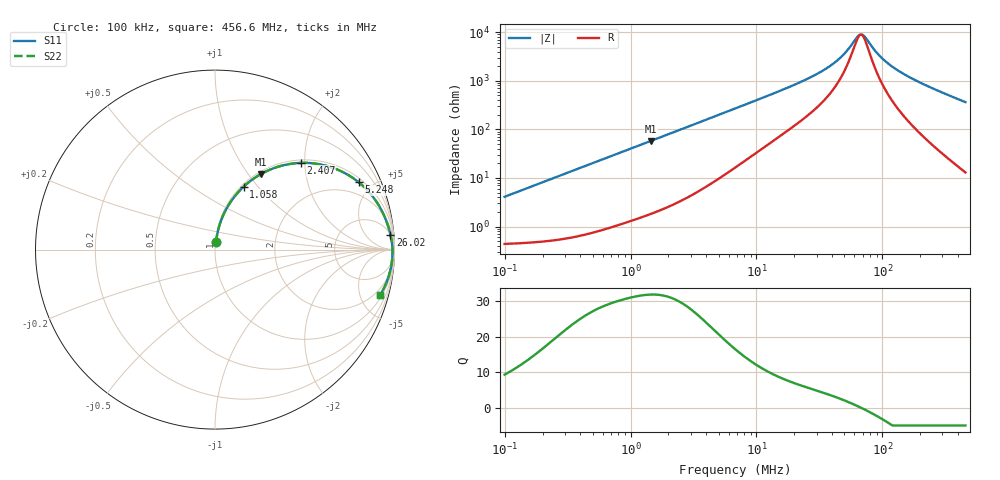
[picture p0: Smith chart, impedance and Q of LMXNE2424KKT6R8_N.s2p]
! LMXNE2424KKT6R8_N  S-PARAMETER MODEL  ( General Type )
! Model Generated by TAIYO YUDEN Corporation (https://www.yuden.co.jp/en/)
! Version 1.0
! TAIYO YUDEN Control No. 191023NI43SB-FBB
! Copyright(c) 2019 TAIYO YUDEN CO.,LTD. All Rights Reserved.
! Product Description (link to TY-COMPAS)
! https://ds.yuden.co.jp/TYCOMPAS/or/detail?pn=LMXNE2424KKT6R8MN&u=M
! Products Name : Inductors
! Characteristics :
!  Inductance : 6.8 uH , SRF(min) : 43 MHz , DC Resistance(max) : 0.492 Ohm
!  Rated Current : Saturation :750 mA , Temp Rise : 570 mA (40 degC)
!  Case Size : 2.4 x 2.4 / 0.095 x 0.095 [mm/inch] , Thickness : 1 / 0.039 [mm/inch]
!  (Conditions: Temperature = 25 degC , DC Bias Current/Voltage = 0A / 0V)
! External Node Assignments :
!  1  o---GGG---o  2
! GND o---------o GND
! Frequency Range : 0.1MHz  -  456.598367MHz  [ 402 STEP ]
# MHz S RI R 50
! Freq[MHz].  S11 Real  S11 Imag  S21 Real  S21 Imag  S12 Real  S12 Imag  S22 Real  S22 Imag
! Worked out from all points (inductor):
!   401 points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, 100 kHz to 456.6 MHz, reference 50 ohm
!   read as one part in series: L = 6.47 uH near 104.3 kHz
!   highest Q = 31.8 at 1.452 MHz (marker M1), where L = 6.34 uH
!   self-resonance near 67.14 MHz
!   S11 on the Smith chart (normalised r, x): 100 kHz: 1.01, +0.08; 1.058 MHz: 1.03, +0.85; 2.407 MHz: 1.06, +1.91; 5.248 MHz: 1.21, +4.15; 26.02 MHz: 5, +22; 456.6 MHz: 1.26, -7.27
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0.1  0.006 0.0403  0.994 -0.0403  0.994 -0.0403  0.006 0.0403
0.410178  0.0327 0.1593  0.9673 -0.1593  0.9673 -0.1593  0.0327 0.1593
0.694533  0.0797 0.2544  0.9203 -0.2544  0.9203 -0.2544  0.0797 0.2544
1.058448  0.1597 0.3506  0.8403 -0.3506  0.8403 -0.3506  0.1597 0.3506
1.451785  0.2572 0.4216  0.7428 -0.4216  0.7428 -0.4216  0.2572 0.4216
1.682457  0.3147 0.4489  0.6853 -0.4489  0.6853 -0.4489  0.3147 0.4489
2.40699  0.4777 0.4831  0.5223 -0.4831  0.5223 -0.4831  0.4777 0.4831
3.443534  0.6452 0.4596  0.3548 -0.4596  0.3548 -0.4596  0.6452 0.4596
5.247847  0.8003 0.3755  0.1997 -0.3755  0.1997 -0.3755  0.8003 0.3755
6.901063  0.8675 0.3096  0.1325 -0.3096  0.1325 -0.3096  0.8675 0.3096
11.93399  0.9408 0.1927  0.0592 -0.1927  0.0592 -0.1927  0.9408 0.1927
26.01912  0.9773 0.0839  0.0227 -0.0839  0.0227 -0.0839  0.9773 0.0839
27.71655  0.9788 0.0773  0.0212 -0.0773  0.0212 -0.0773  0.9788 0.0773
44.05686  0.9862 0.0347  0.0138 -0.0347  0.0138 -0.0347  0.9862 0.0347
52.14399  0.9877 0.0208  0.0123 -0.0208  0.0123 -0.0208  0.9877 0.0208
63.02949  0.9888 0.0055  0.0112 -0.0055  0.0112 -0.0055  0.9888 0.0055
67.14138  0.989 0.000441  0.011 -0.000441  0.011 -0.000441  0.989 0.000441
73.04418  0.9892 -0.00634  0.0108 0.00634  0.0108 0.00634  0.9892 -0.00634
92.0922  0.989 -0.0255  0.011 0.0255  0.011 0.0255  0.989 -0.0255
113.6871  0.988 -0.0441  0.012 0.0441  0.012 0.0441  0.988 -0.0441
196.5988  0.9794 -0.1034  0.0206 0.1034  0.0206 0.1034  0.9794 -0.1034
456.5984  0.922 -0.251  0.078 0.251  0.078 0.251  0.922 -0.251
